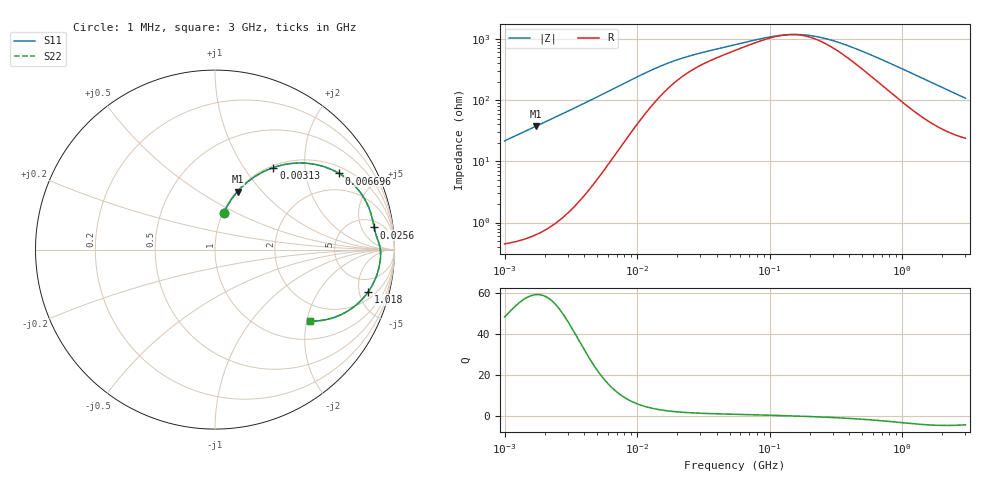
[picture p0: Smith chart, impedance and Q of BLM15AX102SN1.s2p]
! BLM15AX102SN1
# Hz S RI R 50
!Freq.(Hz) S11(Real) S11(Imag) S21(Real) S21(Imag) S12(Real) S12(Imag) S22(Real) S22(Imag)
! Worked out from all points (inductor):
!   401 points, 1 MHz to 3 GHz, reference 50 ohm
!   read as one part in series: L = 3.44 uH near 1.041 MHz
!   highest Q = 59 at 1.717 MHz (marker M1), where L = 3.45 uH
!   self-resonance near 140 MHz
!   S11 on the Smith chart (normalised r, x): 1 MHz: 1.01, +0.43; 3.13 MHz: 1.03, +1.38; 6.696 MHz: 1.24, +3.08; 25.6 MHz: 7, +9; 1.018 GHz: 2.80, -6.11; 3 GHz: 1.48, -2.09
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1000000  0.0484 0.2045  0.9516 -0.2045  0.9516 -0.2045  0.0484 0.2045
1716745  0.1258 0.3233  0.8742 -0.3233  0.8742 -0.3233  0.1258 0.3233
2317916  0.2075 0.3966  0.7925 -0.3966  0.7925 -0.3966  0.2075 0.3966
3129607  0.3249 0.4571  0.6751 -0.4571  0.6751 -0.4571  0.3249 0.4571
3823119  0.4204 0.4792  0.5796 -0.4792  0.5796 -0.4792  0.4204 0.4792
5059610  0.563 0.4735  0.437 -0.4735  0.437 -0.4735  0.563 0.4735
6696013  0.6916 0.4243  0.3084 -0.4243  0.3084 -0.4243  0.6916 0.4243
9600343  0.8047 0.325  0.1953 -0.325  0.1953 -0.325  0.8047 0.325
1.461624e7  0.8639 0.2152  0.1361 -0.2152  0.1361 -0.2152  0.8639 0.2152
2.559965e7  0.8869 0.1235  0.1131 -0.1235  0.1131 -0.1235  0.8869 0.1235
5.477226e7  0.9046 0.0606  0.0954 -0.0606  0.0954 -0.0606  0.9046 0.0606
9.034013e7  0.9157 0.0286  0.0843 -0.0286  0.0843 -0.0286  0.9157 0.0286
1.219755e8  0.92 0.00916  0.08 -0.00916  0.08 -0.00916  0.92 0.00916
1.614254e8  0.9223 -0.00978  0.0777 0.00978  0.0777 0.00978  0.9223 -0.00978
2.094008e8  0.9228 -0.0287  0.0772 0.0287  0.0772 0.0287  0.9228 -0.0287
2.662515e8  0.9218 -0.0482  0.0782 0.0482  0.0782 0.0482  0.9218 -0.0482
3.523638e8  0.9186 -0.0746  0.0814 0.0746  0.0814 0.0746  0.9186 -0.0746
8.005644e8  0.8812 -0.1892  0.1188 0.1892  0.1188 0.1892  0.8812 -0.1892
1.017911e9  0.8531 -0.236  0.1469 0.236  0.1469 0.236  0.8531 -0.236
1.645649e9  0.75 -0.3358  0.25 0.3358  0.25 0.3358  0.75 -0.3358
2.266846e9  0.6409 -0.3848  0.3591 0.3848  0.3591 0.3848  0.6409 -0.3848
3e9  0.529 -0.3982  0.471 0.3982  0.471 0.3982  0.529 -0.3982
